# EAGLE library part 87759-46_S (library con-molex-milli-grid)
HEADER
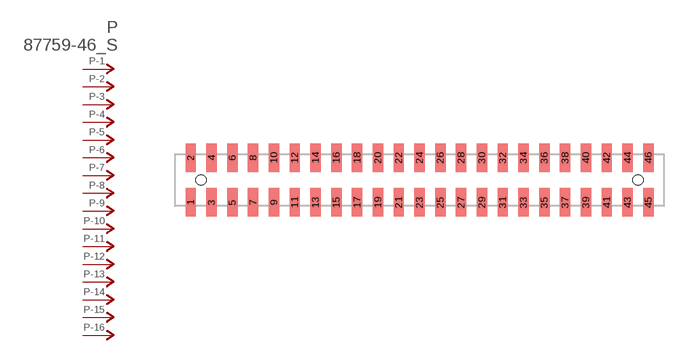
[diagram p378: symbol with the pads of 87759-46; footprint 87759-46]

Designator prefix P; gates -1=P-NV -2=P-N -3=P-N -4=P-N -5=P-N -6=P-N -7=P-N -8=P-N -9=P-N -10=P-N -11=P-N -12=P-N -13=P-N -14=P-N -15=P-N -16=P-N -17=P-N -18=P-N -19=P-N -20=P-N -21=P-N -22=P-N -23=P-N -24=P-N -25=P-N -26=P-N -27=P-N -28=P-N -29=P-N -30=P-N -31=P-N -32=P-N -33=P-N -34=P-N -35=P-N -36=P-N -37=P-N -38=P-N -39=P-N -40=P-N -41=P-N -42=P-N -43=P-N -44=P-N -45=P-N -46=P-N

## 87759-46_S  [87759-46]
1  -1:P  pas
2  -2:P  pas
3  -3:P  pas
4  -4:P  pas
5  -5:P  pas
6  -6:P  pas
7  -7:P  pas
8  -8:P  pas
9  -9:P  pas
10  -10:P  pas
11  -11:P  pas
12  -12:P  pas
13  -13:P  pas
14  -14:P  pas
15  -15:P  pas
16  -16:P  pas
17  -17:P  pas
18  -18:P  pas
19  -19:P  pas
20  -20:P  pas
21  -21:P  pas
22  -22:P  pas
23  -23:P  pas
24  -24:P  pas
25  -25:P  pas
26  -26:P  pas
27  -27:P  pas
28  -28:P  pas
29  -29:P  pas
30  -30:P  pas
31  -31:P  pas
32  -32:P  pas
33  -33:P  pas
34  -34:P  pas
35  -35:P  pas
36  -36:P  pas
37  -37:P  pas
38  -38:P  pas
39  -39:P  pas
40  -40:P  pas
41  -41:P  pas
42  -42:P  pas
43  -43:P  pas
44  -44:P  pas
45  -45:P  pas
46  -46:P  pas

## Footprint 87759-46 (pad centres in mm)
HEADER SMD Dual Row, Vertical
smd 1 x 2.75: 1 -22,-2.15; 2 -22,2.15; 3 -20,-2.15; 4 -20,2.15; 5 -18,-2.15; 6 -18,2.15; 7 -16,-2.15; 8 -16,2.15; 9 -14,-2.15; 10 -14,2.15; 11 -12,-2.15; 12 -12,2.15; 13 -10,-2.15; 14 -10,2.15; 15 -8,-2.15; 16 -8,2.15; 17 -6,-2.15; 18 -6,2.15; 19 -4,-2.15; 20 -4,2.15; 21 -2,-2.15; 22 -2,2.15; 23 0,-2.15; 24 0,2.15; 25 2,-2.15; 26 2,2.15; 27 4,-2.15; 28 4,2.15; 29 6,-2.15; 30 6,2.15; 31 8,-2.15; 32 8,2.15; 33 10,-2.15; 34 10,2.15; 35 12,-2.15; 36 12,2.15; 37 14,-2.15; 38 14,2.15; 39 16,-2.15; 40 16,2.15; 41 18,-2.15; 42 18,2.15; 43 20,-2.15; 44 20,2.15; 45 22,-2.15; 46 22,2.15
hole 1 at -21,0
hole 1 at 21,0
